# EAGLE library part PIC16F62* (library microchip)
FLASH-Based 8-Bit CMOS Microcontroller Source: http://ww1.microchip.com/downloads/en/DeviceDoc/40300C.pdf
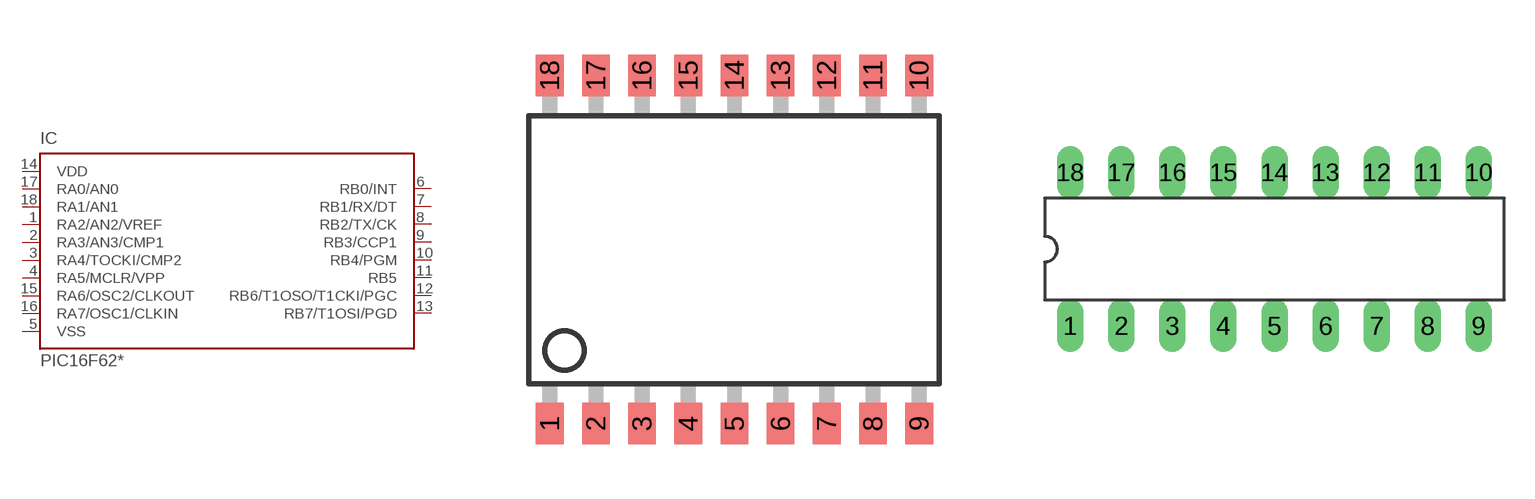
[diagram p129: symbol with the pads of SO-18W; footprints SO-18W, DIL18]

Designator prefix IC

## PIC16F627SO (MF: MICROCHIP; MPN: PIC16F627-04I/SO; OC_FARNELL: 9760296; OC_NEWARK: 19C7271), PIC16F628SO (MF: MICROCHIP; MPN: PIC16F628-20I/SO; OC_FARNELL: 9760415; OC_NEWARK: 23C4986)  [SO-18W]
1  RA2/AN2/VREF
2  RA3/AN3/CMP1
3  RA4/TOCKI/CMP2
4  RA5/MCLR/VPP
5  VSS  pwr
6  RB0/INT
7  RB1/RX/DT
8  RB2/TX/CK
9  RB3/CCP1
10  RB4/PGM
11  RB5
12  RB6/T1OSO/T1CKI/PGC
13  RB7/T1OSI/PGD
14  VDD  pwr
15  RA6/OSC2/CLKOUT
16  RA7/OSC1/CLKIN
17  RA0/AN0
18  RA1/AN1

## PIC16F627P (MF: MICROCHIP; MPN: PIC16F627-04/P; OC_FARNELL: 1084298; OC_NEWARK: 23C4960), PIC16F628P (MF: MICROCHIP; MPN: PIC16F628-04I/P; OC_FARNELL: 9760407; OC_NEWARK: 19C7272)  [DIL18]
Pads as for SO-18W

## Footprint SO-18W (pad centres in mm)
Small Outline Wide Plastic Gull Wing 300-mil body, package type SO
smd 0.762 x 1.143: 1 -5.08,-4.788; 2 -3.81,-4.788; 3 -2.54,-4.788; 4 -1.27,-4.788; 5 0,-4.788; 6 1.27,-4.788; 7 2.54,-4.788; 8 3.81,-4.788; 9 5.08,-4.788; 10 5.08,4.788; 11 3.81,4.788; 12 2.54,4.788; 13 1.27,4.788; 14 0,4.788; 15 -1.27,4.788; 16 -2.54,4.788; 17 -3.81,4.788; 18 -5.08,4.788

## Footprint DIL18 (pad centres in mm)
Dual In Line package type P
drill 0.813 long: 1 -10.16,-3.81; 2 -7.62,-3.81; 3 -5.08,-3.81; 4 -2.54,-3.81; 5 0,-3.81; 6 2.54,-3.81; 7 5.08,-3.81; 8 7.62,-3.81; 9 10.16,-3.81; 10 10.16,3.81; 11 7.62,3.81; 12 5.08,3.81; 13 2.54,3.81; 14 0,3.81; 15 -2.54,3.81; 16 -5.08,3.81; 17 -7.62,3.81; 18 -10.16,3.81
